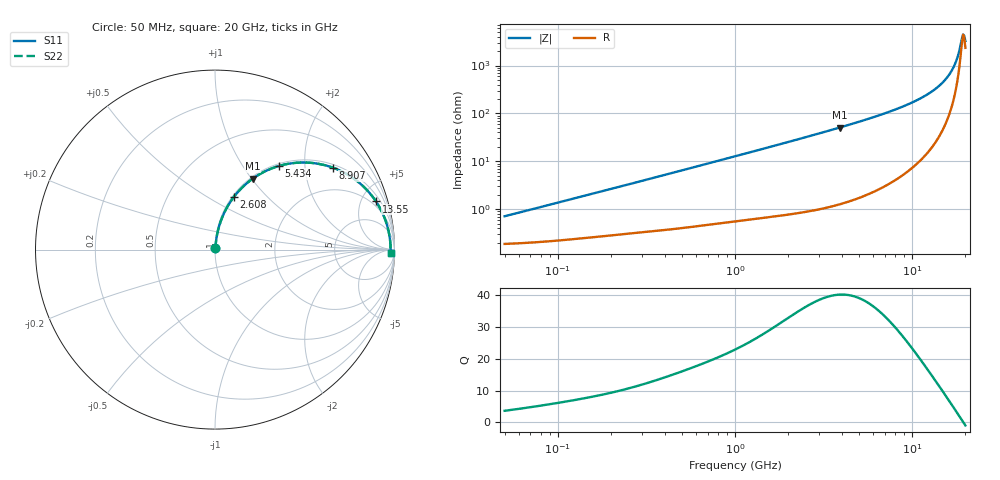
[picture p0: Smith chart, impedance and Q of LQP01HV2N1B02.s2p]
!Murata Part Number: LQP01HV2N1B02
!These Parameters are Measured in Series Mode Connection
!  o--[Z]--o
!Port1  Port2
!  o-------o
!Freq. Start=50[MHz] Stop=20[GHz], 401[Steps]
# Hz S RI R 50
!Freq.(Hz) S11(Real) S11(Imag) S21(Real) S21(Imag) S12(Real) S12(Imag) S22(Real) S22(Imag)
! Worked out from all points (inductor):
!   401 points, 50 MHz to 20 GHz, reference 50 ohm
!   read as one part in series: L = 2.18 nH near 51.52 MHz
!   highest Q = 40.2 at 3.908 GHz (marker M1), where L = 2.07 nH
!   self-resonance near 19.41 GHz
!   S11 on the Smith chart (normalised r, x): 50 MHz: 1.00, +0.01; 2.608 GHz: 1.02, +0.66; 5.434 GHz: 1.04, +1.47; 8.907 GHz: 1.10, +2.81; 13.55 GHz: 1.50, +6.50; 20 GHz: 48, -45
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5e7  0.00192 0.00684  0.9981 -0.00684  0.9981 -0.00684  0.00192 0.00684
1.364002e8  0.00278 0.0182  0.9972 -0.0182  0.9972 -0.0182  0.00278 0.0182
3.721004e8  0.00584 0.0478  0.9942 -0.0478  0.9942 -0.0478  0.00584 0.0478
1e9  0.0211 0.1237  0.9789 -0.1237  0.9789 -0.1237  0.0211 0.1237
1.714689e9  0.0512 0.2045  0.9488 -0.2045  0.9488 -0.2045  0.0512 0.2045
2.608132e9  0.1059 0.2945  0.8941 -0.2945  0.8941 -0.2945  0.1059 0.2945
2.728004e9  0.1145 0.3054  0.8855 -0.3054  0.8855 -0.3054  0.1145 0.3054
3.908127e9  0.2113 0.396  0.7887 -0.396  0.7887 -0.396  0.2113 0.396
5.433528e9  0.3545 0.4654  0.6455 -0.4654  0.6455 -0.4654  0.3545 0.4654
7.442007e9  0.5402 0.483  0.4598 -0.483  0.4598 -0.483  0.5402 0.483
8.907419e9  0.6578 0.4562  0.3422 -0.4562  0.3422 -0.4562  0.6578 0.4562
1.131968e10  0.8069 0.3696  0.1931 -0.3696  0.1931 -0.3696  0.8069 0.3696
1.354865e10  0.8971 0.268  0.1029 -0.268  0.1029 -0.268  0.8971 0.268
1.527346e10  0.9408 0.1863  0.0592 -0.1863  0.0592 -0.1863  0.9408 0.1863
1.670968e10  0.9631 0.1197  0.0369 -0.1197  0.0369 -0.1197  0.9631 0.1197
1.721783e10  0.9684 0.0968  0.0316 -0.0968  0.0316 -0.0968  0.9684 0.0968
1.774144e10  0.9726 0.0736  0.0274 -0.0736  0.0274 -0.0736  0.9726 0.0736
1.828096e10  0.9756 0.0503  0.0244 -0.0503  0.0244 -0.0503  0.9756 0.0503
1.88369e10  0.9775 0.0268  0.0225 -0.0268  0.0225 -0.0268  0.9775 0.0268
1.912117e10  0.9781 0.015  0.0219 -0.015  0.0219 -0.015  0.9781 0.015
1.970266e10  0.9783 -0.00859  0.0217 0.00859  0.0217 0.00859  0.9783 -0.00859
2e10  0.978 -0.0204  0.022 0.0204  0.022 0.0204  0.978 -0.0204
